(* Logix 5000 DataType export A1000_OUT; software revision 20.05 *)

TYPE A1000_CONTROL :
STRUCT
   TriggerEnable : BOOL;
   BufferResultsEnable : BOOL;
   reserved_0_2 : BOOL;
   reserved_0_3 : BOOL;
   ExecuteCommand : BOOL;
   reserved_0_5 : BOOL;
   ClearError : BOOL;
   reserved_0_7 : BOOL;
   CommandID : INT;
   SoftEvent0 : BOOL;
   SoftEvent1 : BOOL;
   SoftEvent2 : BOOL;
   SoftEvent3 : BOOL;
   SoftEvent4 : BOOL;
   SoftEvent5 : BOOL;
   SoftEvent6 : BOOL;
   SoftEvent7 : BOOL;
   SoftEvent8 : BOOL;
   SoftEvent9 : BOOL;
   SoftEvent10 : BOOL;
   SoftEvent11 : BOOL;
   SoftEvent12 : BOOL;
   SoftEvent13 : BOOL;
   SoftEvent14 : BOOL;
   SoftEvent15 : BOOL;
   SoftEvent16 : BOOL;
   SoftEvent17 : BOOL;
   SoftEvent18 : BOOL;
   SoftEvent19 : BOOL;
   SoftEvent20 : BOOL;
   SoftEvent21 : BOOL;
   SoftEvent22 : BOOL;
   SoftEvent23 : BOOL;
   SoftEvent24 : BOOL;
   SoftEvent25 : BOOL;
   SoftEvent26 : BOOL;
   SoftEvent27 : BOOL;
   SoftEvent28 : BOOL;
   SoftEvent29 : BOOL;
   SoftEvent30 : BOOL;
   SoftEvent31 : BOOL;
   TriggerCamera0 : BOOL;
   InspectionResultsAck0 : BOOL;
   ClearExposureComplete0 : BOOL;
   SetUserData0 : BOOL;
   reserved_16_4 : BOOL;
   reserved_16_5 : BOOL;
   reserved_16_6 : BOOL;
   reserved_16_7 : BOOL;
   TriggerCamera1 : BOOL;
   InspectionResultsAck1 : BOOL;
   ClearExposureComplete1 : BOOL;
   SetUserData1 : BOOL;
   reserved_17_4 : BOOL;
   reserved_17_5 : BOOL;
   reserved_17_6 : BOOL;
   reserved_17_7 : BOOL;
   TriggerCamera2 : BOOL;
   InspectionResultsAck2 : BOOL;
   ClearExposureComplete2 : BOOL;
   SetUserData2 : BOOL;
   reserved_18_4 : BOOL;
   reserved_18_5 : BOOL;
   reserved_18_6 : BOOL;
   reserved_18_7 : BOOL;
   TriggerCamera3 : BOOL;
   InspectionResultsAck3 : BOOL;
   ClearExposureComplete3 : BOOL;
   SetUserData3 : BOOL;
   reserved_19_4 : BOOL;
   reserved_19_5 : BOOL;
   reserved_19_6 : BOOL;
   reserved_19_7 : BOOL;
END_STRUCT
END_TYPE

TYPE A1000_OUT :
STRUCT
   Control : A1000_CONTROL;
   UserData : SINT[480];
END_STRUCT
END_TYPE
